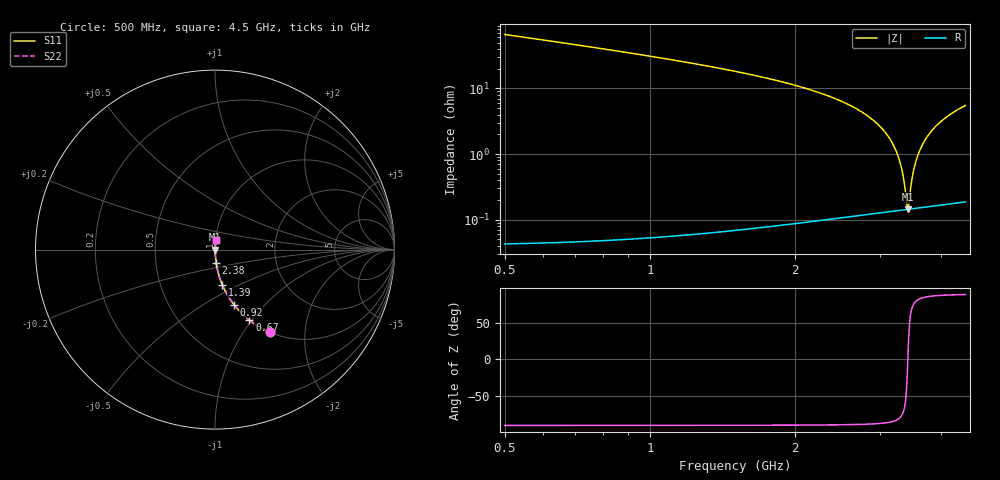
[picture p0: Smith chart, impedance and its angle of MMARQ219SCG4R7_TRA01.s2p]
! MMARQ219SCG4R7_TRA01  S-PARAMETER MODEL  ( General Type )
! Model Generated by TAIYO YUDEN Corporation (http://www.ty-top.com)
! Version 1.0
! TAIYO YUDEN Control No. 160201
! Copyright(c) 2016 TAIYO YUDEN CO.,LTD. All Rights Reserved.
! Product Description (link to TY-COMPAS)
! https://ds.yuden.co.jp/TYCOMPAS/or/detail?pn=MMARQ219SCG4R7BTRA01&u=M
! Products Name : Multilayer Ceramic Capacitors
! Characteristics :
!  Capacitance : 4.7 pF , Rated Voltage : 250V , TCC : CG / C0G
!  Case Size : 2.0 x 1.25 / 0.079 x 0.049 [mm/inch] , Thickness : 0.85 / 0.033 [mm/inch]
!  (Conditions: Temperature = 25 degC , DC Bias Current/Voltage = 0A / 0V)
! External Node Assignments :
!  1  o---| |---o  2
! GND o---------o GND
! Frequency Range : 500MHz  -  4500MHz  [ 401 STEP ]
# MHz S RI R 50
! Freq[MHz].  S11 Real  S11 Imag  S21 Real  S21 Imag  S12 Real  S12 Imag  S22 Real  S22 Imag
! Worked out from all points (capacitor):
!   401 points, 500 MHz to 4.5 GHz, reference 50 ohm
!   read as one part in series: C = 4.69 pF near 520 MHz
!   lowest |Z| = 144 mohm at 3.42 GHz (marker M1)
!   series resonance near 3.42 GHz, so ESL is about 460 pH
!   S11 on the Smith chart (normalised r, x): 500 MHz: 1.00, -1.33; 670 MHz: 1.00, -0.97; 920 MHz: 1.00, -0.68; 1.39 GHz: 1.00, -0.41; 2.38 GHz: 1.00, -0.15; 4.5 GHz: 1.00, +0.11
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500  0.3064 -0.4607  0.6936 0.4607  0.6936 0.4607  0.3064 -0.4607
670  0.192 -0.3934  0.808 0.3934  0.808 0.3934  0.192 -0.3934
920  0.1052 -0.306  0.8948 0.306  0.8948 0.306  0.1052 -0.306
1170  0.062 -0.24  0.938 0.24  0.938 0.24  0.062 -0.24
1390  0.0404 -0.1953  0.9596 0.1953  0.9596 0.1953  0.0404 -0.1953
1840  0.0176 -0.1285  0.9824 0.1285  0.9824 0.1285  0.0176 -0.1285
2380  0.00636 -0.0728  0.9936 0.0728  0.9936 0.0728  0.00636 -0.0728
2500  0.00502 -0.0627  0.995 0.0627  0.995 0.0627  0.00502 -0.0627
2910  0.00226 -0.032  0.9977 0.032  0.9977 0.032  0.00226 -0.032
3170  0.00156 -0.015  0.9984 0.015  0.9984 0.015  0.00156 -0.015
3250  0.00147 -0.0101  0.9985 0.0101  0.9985 0.0101  0.00147 -0.0101
3310  0.00144 -0.00644  0.9986 0.00644  0.9986 0.00644  0.00144 -0.00644
3350  0.00143 -0.00407  0.9986 0.00407  0.9986 0.00407  0.00143 -0.00407
3400  0.00143 -0.00114  0.9986 0.00114  0.9986 0.00114  0.00143 -0.00114
3420  0.00144 1.21e-05  0.9986 -1.21e-05  0.9986 -1.21e-05  0.00144 1.21e-05
3440  0.00145 0.00116  0.9986 -0.00116  0.9986 -0.00116  0.00145 0.00116
3500  0.00149 0.00457  0.9985 -0.00457  0.9985 -0.00457  0.00149 0.00457
3570  0.00157 0.00848  0.9984 -0.00848  0.9984 -0.00848  0.00157 0.00848
3680  0.00175 0.0145  0.9982 -0.0145  0.9982 -0.0145  0.00175 0.0145
3840  0.00213 0.0229  0.9979 -0.0229  0.9979 -0.0229  0.00213 0.0229
4120  0.00307 0.0369  0.9969 -0.0369  0.9969 -0.0369  0.00307 0.0369
4500  0.00485 0.0545  0.9951 -0.0545  0.9951 -0.0545  0.00485 0.0545
